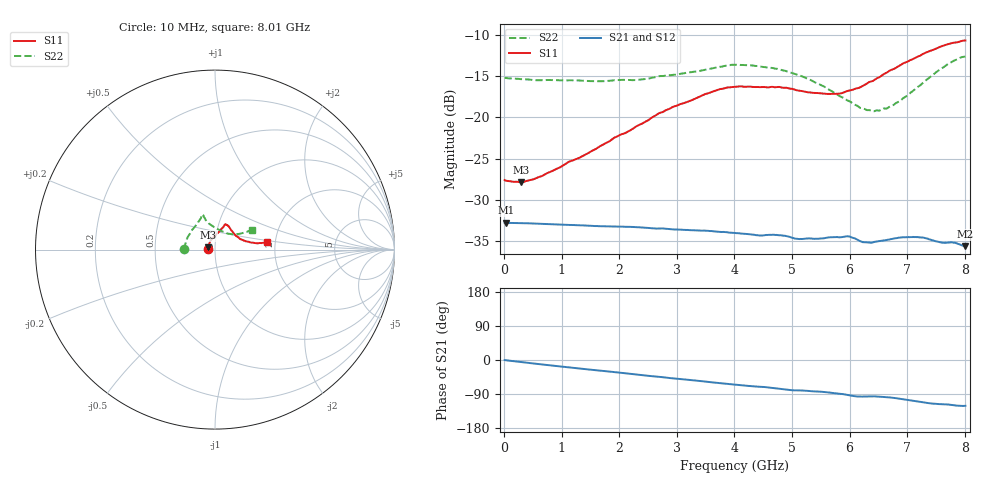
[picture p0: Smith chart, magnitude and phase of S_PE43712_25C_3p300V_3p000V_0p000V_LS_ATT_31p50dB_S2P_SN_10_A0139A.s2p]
! DEVICE ID: PE43712
! File Path: z:\PE43713\PE43713_CHAR_NOM_04292014\AMB\3p300\LS_ATT_31p50dB\PE43713_AMB_3p300V_3p000V_0p000V_LS_ATT_31p50dB_S2P_SN_10_A0139A.s2p
! Serial: 10
! Lot: A0139A
! Temp: 25C
! VDD: 3.300
! VSS: 0.000
! Control_Hi: 3.000
! Control_Lo: 0.000
! Attenuation Step: 31.50dB
! Port 1: RF1
! Port 2: RF2
! ThroughPath:1-2
! IDD: 0.0001459154
! ISS: -6.23e-008
#  Hz  S  RI  R  50
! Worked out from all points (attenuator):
!   801 points, 10 MHz to 8.01 GHz, reference 50 ohm
!   highest |S21| = -32.78 dB at 30 MHz (marker M1); lowest = -35.6 dB at 8.01 GHz (marker M2)
!   lowest |S11| = -27.9 dB at 290 MHz (marker M3), VSWR 1.08, Z = 46.3 + j1.23 ohm
!   |S11| at or under -10 dB: start of sweep to end of sweep
!   |S22| runs from -19.3 to -12.6 dB; largest |S21 - S12| = 0.0001
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1e7  -0.0417 0.000872  0.023 -0.000107  0.023 -7.23e-05  -0.1734 0.00116
3e7  -0.0412 0.00222  0.023 -0.000233  0.023 -0.000242  -0.1728 0.00285
2.9e8  -0.0381 0.0133  0.0228 -0.0021  0.0228 -0.00211  -0.1693 0.018
6.5e8  -0.0338 0.0282  0.0222 -0.00452  0.0222 -0.00452  -0.1631 0.0382
1.35e9  -0.021 0.054  0.0204 -0.00872  0.0204 -0.00871  -0.149 0.0744
2.31e9  0.0103 0.0881  0.0169 -0.0134  0.0169 -0.0134  -0.115 0.1228
2.68e9  0.025 0.1024  0.0152 -0.0148  0.0152 -0.0148  -0.0997 0.1464
3.5e9  0.0484 0.1298  0.0112 -0.0172  0.0112 -0.0172  -0.0774 0.178
3.74e9  0.0533 0.138  0.00984 -0.0177  0.00986 -0.0177  -0.0755 0.1874
4.01e9  0.0582 0.1416  0.00842 -0.0181  0.00842 -0.018  -0.075 0.1941
4.76e9  0.0722 0.1345  0.00479 -0.0187  0.00482 -0.0188  -0.0624 0.1858
5.09e9  0.0821 0.1201  0.00313 -0.0181  0.00316 -0.0181  -0.0553 0.1727
5.35e9  0.0912 0.1073  0.00239 -0.0183  0.00241 -0.0182  -0.0485 0.1592
5.77e9  0.1114 0.0826  0.00056 -0.0188  0.000592 -0.0188  -0.0216 0.1367
5.96e9  0.125 0.0719  -0.000651 -0.019  -0.000635 -0.019  -0.00652 0.1264
6.2e9  0.1414 0.0584  -0.00203 -0.0176  -0.00199 -0.0176  0.0179 0.1123
6.41e9  0.1583 0.0514  -0.00183 -0.0174  -0.0018 -0.0174  0.0408 0.1006
6.68e9  0.1852 0.0435  -0.00273 -0.018  -0.00271 -0.018  0.0724 0.0895
6.87e9  0.2017 0.039  -0.00392 -0.0183  -0.00392 -0.0183  0.0911 0.0858
7.22e9  0.233 0.0354  -0.00645 -0.0176  -0.00641 -0.0176  0.1291 0.0871
7.7e9  0.274 0.0391  -0.00797 -0.0155  -0.008 -0.0155  0.1835 0.1014
8.01e9  0.2887 0.0432  -0.00851 -0.0142  -0.00849 -0.0142  0.2057 0.1098
